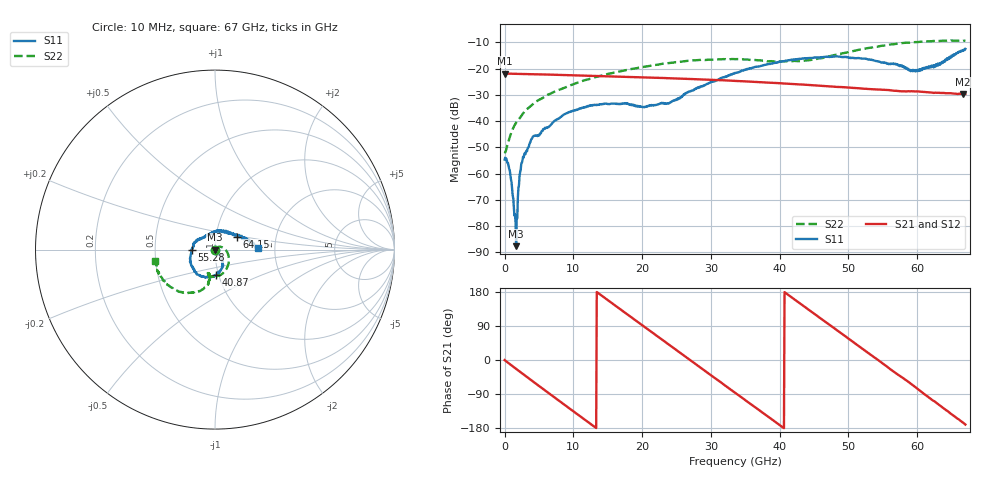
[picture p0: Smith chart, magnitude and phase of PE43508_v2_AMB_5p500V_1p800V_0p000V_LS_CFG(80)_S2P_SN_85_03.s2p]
!Keysight Technologies,N5227A,US51270237,A.10.43.00
!Date: Wednesday, August 22, 2018 17:14:59
!Correction: S11(Full 2 Port(1,3))
!S31(Full 2 Port(1,3))
!S13(Full 2 Port(1,3))
!S33(Full 2 Port(1,3))
!S2P File: Measurements: S11, S31, S13, S33:
# Hz S  dB  R 50
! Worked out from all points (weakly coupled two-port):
!   801 points, 10 MHz to 67 GHz, reference 50 ohm
!   highest |S21| = -21.88 dB at 10 MHz (marker M1); lowest = -29.7 dB at 66.67 GHz (marker M2)
!   lowest |S11| = -87.6 dB at 1.685 GHz (marker M3), VSWR 1.00, Z = 50 - j0.00129 ohm
!   |S11| at or under -10 dB: start of sweep to end of sweep
!   |S22| runs from -52.0 to -9.3 dB; largest |S21 - S12| = 0.00038
!   S11 on the Smith chart (normalised r, x): 10 MHz: 1.00, -0.00; 40.87 GHz: 0.97, -0.28; 55.28 GHz: 0.77, +0.00; 64.15 GHz: 1.27, +0.19; 67 GHz: 1.62, +0.03
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1e7  -54.66 -168.6  -21.88 -0.3  -21.88 -0.2  -51.67 -3.3
6.799e8  -58.25 175.0  -21.94 -9.6  -21.95 -9.6  -46.70 44.7
1.433538e9  -75.99 160.8  -21.99 -20.0  -21.99 -20.0  -41.70 51.7
1.68475e9  -87.63 -161.8  -22.01 -23.5  -22.00 -23.5  -40.59 53.0
1.935962e9  -69.10 -67.1  -22.02 -26.9  -22.02 -26.9  -39.77 53.0
2.270912e9  -59.38 -59.0  -22.04 -31.5  -22.04 -31.5  -38.69 51.0
2.522125e9  -55.88 -46.6  -22.05 -34.9  -22.05 -34.9  -37.75 49.6
4.0294e9  -46.34 -40.9  -22.15 -55.3  -22.15 -55.3  -33.77 41.5
8.634962e9  -37.52 -68.9  -22.44 -117.1  -22.43 -117.1  -27.38 16.1
1.123082e10  -34.94 -77.2  -22.62 -151.7  -22.63 -151.7  -24.83 -0.4
2.236791e10  -33.54 -72.1  -23.54 60.7  -23.53 60.7  -18.47 -55.3
2.395892e10  -33.11 -59.9  -23.68 39.7  -23.68 39.7  -17.87 -61.8
3.3505e10  -21.75 -58.9  -24.70 -86.4  -24.70 -86.4  -16.39 -97.5
4.08739e10  -16.99 -87.5  -25.72 176.8  -25.72 176.8  -17.18 -105.7
4.472582e10  -15.94 -107.0  -26.31 126.0  -26.29 126.1  -16.67 -101.2
4.841028e10  -15.36 -126.5  -26.99 77.6  -26.99 77.5  -14.68 -100.7
5.527675e10  -17.71 179.8  -28.11 -13.1  -28.08 -13.5  -11.19 -119.5
5.586291e10  -18.33 172.8  -28.18 -21.3  -28.18 -21.7  -10.92 -121.7
6.004979e10  -20.42 107.7  -28.70 -76.0  -28.71 -76.5  -9.90 -138.7
6.415292e10  -16.86 30.4  -29.39 -131.8  -29.45 -132.1  -9.39 -156.1
6.666505e10  -13.27 5.9  -29.67 -165.4  -29.75 -165.4  -9.42 -167.4
6.7e10  -12.49 1.9  -29.66 -170.3  -29.73 -170.3  -9.40 -169.2
